(* 	
	Program Name: 	ACS_WRITE_AXIS_VARIABLES
	Purpose:		(To be used only by Output Scan Function) Copy Drive Variables from shadow memory to output registers 
*)
PROGRAM ACS_WRITE_AXIS_VARIABLES
VAR_IN_OUT
	Axis:ACS_DRIVE_TYPE;
END_VAR

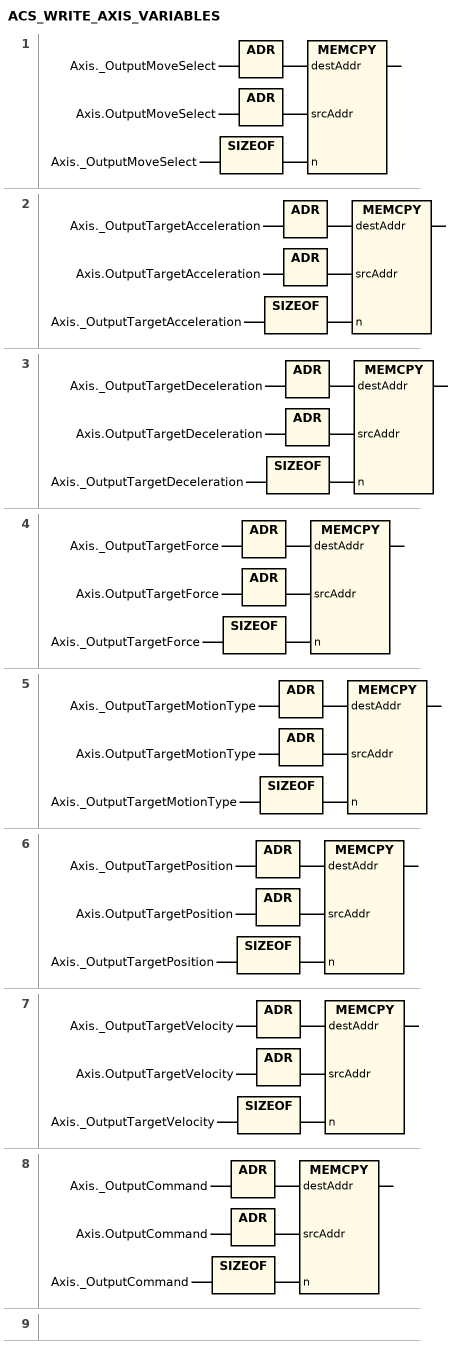
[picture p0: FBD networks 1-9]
// NETWORK 1
MEMCPY(destAddr := ADR(Axis._OutputMoveSelect), srcAddr := ADR(Axis.OutputMoveSelect), n := SIZEOF(Axis._OutputMoveSelect));

// NETWORK 2
MEMCPY(destAddr := ADR(Axis._OutputTargetAcceleration), srcAddr := ADR(Axis.OutputTargetAcceleration), n := SIZEOF(Axis._OutputTargetAcceleration));

// NETWORK 3
MEMCPY(destAddr := ADR(Axis._OutputTargetDeceleration), srcAddr := ADR(Axis.OutputTargetDeceleration), n := SIZEOF(Axis._OutputTargetDeceleration));

// NETWORK 4
MEMCPY(destAddr := ADR(Axis._OutputTargetForce), srcAddr := ADR(Axis.OutputTargetForce), n := SIZEOF(Axis._OutputTargetForce));

// NETWORK 5
MEMCPY(destAddr := ADR(Axis._OutputTargetMotionType), srcAddr := ADR(Axis.OutputTargetMotionType), n := SIZEOF(Axis._OutputTargetMotionType));

// NETWORK 6
MEMCPY(destAddr := ADR(Axis._OutputTargetPosition), srcAddr := ADR(Axis.OutputTargetPosition), n := SIZEOF(Axis._OutputTargetPosition));

// NETWORK 7
MEMCPY(destAddr := ADR(Axis._OutputTargetVelocity), srcAddr := ADR(Axis.OutputTargetVelocity), n := SIZEOF(Axis._OutputTargetVelocity));

// NETWORK 8
MEMCPY(destAddr := ADR(Axis._OutputCommand), srcAddr := ADR(Axis.OutputCommand), n := SIZEOF(Axis._OutputCommand));

// NETWORK 9

END_PROGRAM
